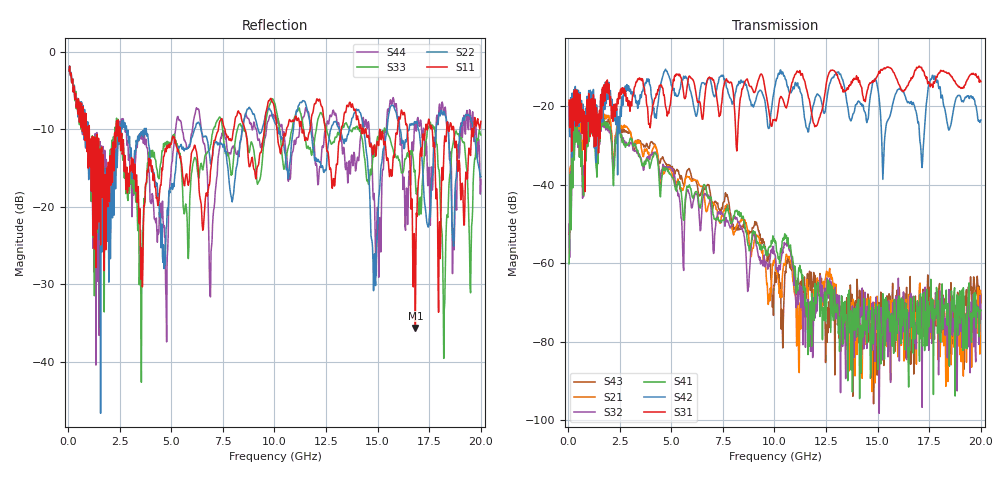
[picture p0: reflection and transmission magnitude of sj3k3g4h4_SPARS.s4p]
! FILE: E:\users\goganessyan\GBX_Backplane\FR408_backplane\1m_OUTBOUND_FEXT\sj3k3g4h4_SPARS.s4p
# MHZ S RI R 50.00
! FREQ  S11  S12  S13  S14
!  S21  S22  S23  S24
!  S31  S32  S33  S34
!  S41  S42  S43  S44
!  REAL  IMAG  REAL  IMAG  REAL  IMAG  REAL  IMAG
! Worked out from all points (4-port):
!   799 points, 50 MHz to 20 GHz, reference 50 ohm
!   strongest paths, dB at 50 MHz, 5.025 GHz, 10.03 GHz, 15.03 GHz, 20 GHz:
!     S31: -18.5, -16.1, -23.4, -11.9, -13.8
!     S42: -19.3, -14.9, -14.9, -16.0, -23.6
!     S41: -60.2, -38.1, -54.8, -87.1, -72.1
!     S32: -50.1, -35.8, -57.7, -71.1, -74.2
!     S21: -52.3, -36.9, -58.9, -74.0, -70.2
!     S43: -52.6, -35.8, -62.3, -78.6, -68.1
!   lowest |S11| = -35.6 dB at 16.82 GHz (marker M1), VSWR 1.03, Z = 48.8 - j1.08 ohm
!   |S11| at or under -10 dB: 1.027 GHz to 2.321 GHz (1.294 GHz wide, 77.3 % of centre); 2.512 GHz to 7.282 GHz (4.77 GHz wide, 97.4 % of centre); 14.43 GHz to 15.96 GHz (1.536 GHz wide, 10.1 % of centre)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
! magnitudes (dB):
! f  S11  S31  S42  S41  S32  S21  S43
! 50 MHz  -2.5  -18.5  -19.3  -60.2  -50.1  -52.3  -52.6
! 325 MHz  -6.1  -23.7  -20.9  -26.4  -26.9  -25.1  -25.6
! 1.7 GHz  -13.3  -19.9  -23.8  -22.9  -23.9  -21.8  -23.5
! 11.85 GHz  -8.0  -23.3  -20.5  -74.0  -84.1  -77.2  -66.1
! 14.85 GHz  -12.0  -13.7  -13.2  -71.8  -76.3  -73.6  -80.1
! 16.82 GHz  -35.6  -10.8  -20.9  -79.3  -75.3  -78.2  -68.4
! 20 GHz  -9.0  -13.8  -23.6  -72.1  -74.2  -70.2  -68.1
